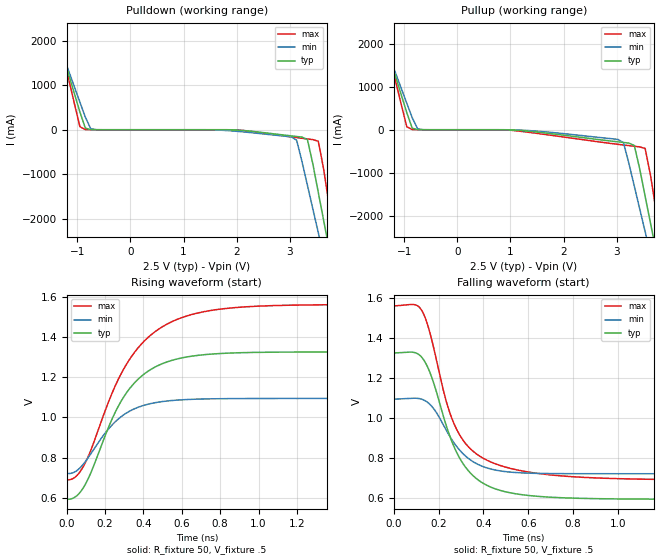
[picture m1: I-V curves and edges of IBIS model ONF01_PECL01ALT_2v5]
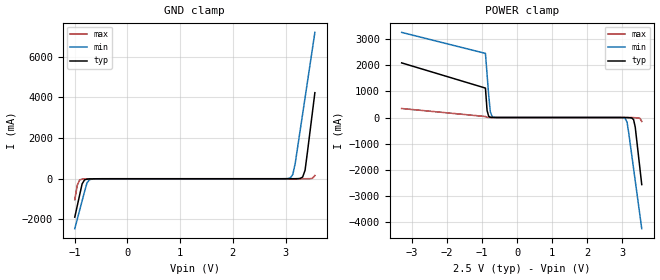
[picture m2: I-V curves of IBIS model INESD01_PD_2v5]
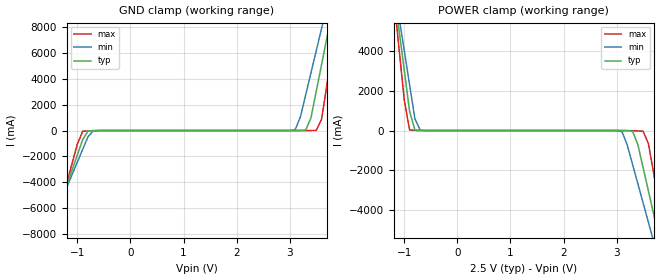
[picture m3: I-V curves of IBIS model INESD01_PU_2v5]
|   This file is an IBIS representation of the   |
|   Integrated Device Technology, Inc.   |
|   8536-02   |
|  Low Skew, 1-to-6, Dual Crystal/LVCMOS-to-3.3V, 2.5V LVPECL Fanout Buffer  |
[IBIS Ver]   4.1
[File name]   8536_02.ibs
[File Rev]   1.0
[Date]   19 Aug 2010
[Source]   Originated at Integrated Device Technology, Inc.
[Disclaimer]
IDT hereby grants the user of this IBIS model a non-exclusive,
nontransferable license to use this IBIS model under the following terms.
Before using this IBIS model, the user should read this license.
If the user does not accept these terms,  the IBIS model should be
returned to IDT within 30 days.
   The user is granted this license only to use the IBIS model and
is not granted rights to sell, load, rent, lease or license the IBIS
model in whole or in part, or in modified form to anyone other than
user. User may modify the IBIS model to suit its specific
applications but rights to derivative works and such modifications
shall belong to IDT.
   This IBIS model is provided on an "AS IS" basis and IDT makes
absolutely no warranty with respect to the information contained
herein. IDT DISCLAIMS AND CUSTOMER WAIVES ALL WARRANTIES, EXPRESS
OR IMPLIED, INCLUDING WARRANTIES OF MERCHANTABILITY OR FITNESS FOR
A PARTICULAR PURPOSE. The entire risk as to quality and performance
is with the Customer. ACCORDINGLY, IN NO EVENT SHALL THE COMPANY BE
LIABLE FOR ANY DAMAGES, WHETHER IN CONTRACT OR TORT,INCLUDING ANY
LOST PROFITS OR OTHER INCIDENTAL, CONSEQUENTIAL, EXEMPLARY, OR
PUNITIVE DAMAGES ARISING OUT OF THE USE OR APPLICATION OF THE IBIS
model provided in this package. Further, IDT reserves the right to
make changes without notice to any product herein to improve
reliability, function, or design. IDT does not convey any license
under patent rights or any other intellectual property rights,
including those of third parties.
   IDT is not obligated to provide maintenance or support
for the licensed IBIS model.
[Copyright]   Copyright 2010 by Integrated Device Technology, Inc.
[Component]   ICS8536G-02
[Manufacturer] Integrated Device Technology, Inc.
[Package]
|TSSOP 24 Lead
|   typ   min   max
R_pkg   60.65m   52.4m   68.9m
L_pkg   1.989nH   1.431nH   2.547nH
C_pkg   0.314pF   0.254pF   0.374pF
[Pin] signal_name  model_name   R_pin   L_pin   C_pin
1   nQ2   ONF01_PECL01ALT   68.9m   2.547n   0.374p
2   Q2   ONF01_PECL01ALT   65.6m   2.323n   0.350p
3   VCC   POWER   62.3m   2.100n   0.326p
4   nQ1   ONF01_PECL01ALT   59.0m   1.877n   0.302p
5   Q1   ONF01_PECL01ALT   55.7m   1.654n   0.278p
6   VEE   GND   52.4m   1.431n   0.254p
7   nQ0   ONF01_PECL01ALT   52.4m   1.431n   0.254p
8   Q0   ONF01_PECL01ALT   55.7m   1.654n   0.278p
9   CLK_SEL0   INESD01_PD   59.0m   1.877n   0.302p
10   XTAL_IN0   NC   62.3m   2.100n   0.326p
11   XTAL_OUT0   NC   65.6m   2.323n   0.350p
12   CLK_EN   INESD01_PU   68.9m   2.547n   0.374p
13   CLK0   INESD02_PD_5V   68.9m   2.547n   0.374p
14   XTAL_IN1   NC   65.6m   2.323n   0.350p
15   XTAL_OUT1   NC   62.3m   2.100n   0.326p
16   CLK_SEL1   INESD01_PD   59.0m   1.877n   0.302p
17   nQ5   ONF01_PECL01ALT   55.7m   1.654n   0.278p
18   Q5   ONF01_PECL01ALT   52.4m   1.431n   0.254p
19   VCC   POWER   52.4m   1.431n   0.254p
20   nQ4   ONF01_PECL01ALT   55.7m   1.654n   0.278p
21   Q4   ONF01_PECL01ALT   59.0m   1.877n   0.302p
22   VCC   POWER   62.3m   2.100n   0.326p
23   nQ3   ONF01_PECL01ALT   65.6m   2.323n   0.350p
24   Q3   ONF01_PECL01ALT   68.9m   2.547n   0.374p
[Diff Pin]  inv_pin  vdiff tdelay_typ tdelay_min  tdelay_max
|Output
2   1   NA   0  0  0
5   4   NA   0  0  0
8   7   NA   0  0  0
18   17   NA   0  0  0
21   20   NA   0  0  0
24   23   NA   0  0  0
[Model Selector] ONF01_PECL01ALT
ONF01_PECL01ALT_2v5  Buffer selection for 2v5
ONF01_PECL01ALT_3v3  Buffer selection for 3v3
[Model Selector] INESD01_PD
INESD01_PD_2v5  Buffer selection for 2v5
INESD01_PD_3v3  Buffer selection for 3v3
[Model Selector] INESD01_PU
INESD01_PU_2v5  Buffer selection for 2v5
INESD01_PU_3v3  Buffer selection for 3v3
[Model Selector] INESD02_PD_5V
INESD02_PD_5V_2v5  Buffer selection for 2v5
INESD02_PD_5V_3v3  Buffer selection for 3v3
| Models and submodels in the file (8): ONF01_PECL01ALT_2v5 (Output_ECL), INESD01_PD_2v5 (Input), INESD01_PU_2v5 (Input), INESD02_PD_5V_2v5 (Input), ONF01_PECL01ALT_3v3 (Output_ECL), INESD01_PD_3v3 (Input), INESD01_PU_3v3 (Input), INESD02_PD_5V_3v3 (Input)
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[Model] ONF01_PECL01ALT_2v5
Model_type  Output_ECL
Polarity   Non-Inverting
Vmeas = .975
Rref = 50
Cref = 0
Vref = .5
|Variable  typ   min   max
C_comp   2p   1.5p   2.5p
[Voltage Range]   2.5   2.375   2.625
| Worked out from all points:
|   rising waveform, R_fixture 50, V_fixture .5: 20-80 % time 228ps typ, 199ps min, 276ps max; typ from 0.592 V to 1.33 V
|   falling waveform, R_fixture 50, V_fixture .5: 20-80 % time 153ps typ, 140ps min, 156ps max; typ from 1.33 V to 0.592 V
| Open source, no load
|  Voltage   I(typ)   I(min)   I(max)
[Pullup]
-3.3V     9.786A     8.425A     12.06A
-1.463V   2.432A     2.308A     2.661A
-952.6mV  398mA      618.5mA    68.87mA
-850.5mV  36.63mA    281.6mA    4.032mA
-646.4mV  229.3uA    964.8uA    177.5uA
3.028V    -282.4mA   -226.8mA   -340.1mA
3.13V     -296.5mA   -301.7mA   -355.4mA
3.334V    -367.3mA   -1.316A    -385.1mA
3.538V    -1.551A    -2.377A    -435.3mA
3.64V     -2.187A    -2.908A    -1.066A
3.844V    -3.46A     -3.969A    -2.688A
6.6V      -20.66A    -18.32A    -24.61A
[Pulldown]
-3.3V     9.786A     8.425A     12.06A
-1.463V   2.432A     2.308A     2.661A
-1.361V   2.024A     1.97A      2.139A
-952.6mV  398mA      618.5mA    68.87mA
-850.5mV  36.63mA    281.6mA    4.032mA
3.028V    -137.6mA   -160.7mA   -160.7mA
3.13V     -151.4mA   -235.1mA   -176.3mA
3.334V    -221.9mA   -1.249A    -206.7mA
3.538V    -1.406A    -2.31A     -257.4mA
3.64V     -2.042A    -2.84A     -888.8mA
3.844V    -3.314A    -3.9A      -2.51A
6.6V      -20.58A    -18.26A    -24.54A
[Ramp]
|   typ   min   max
dV/dt_r   0.586/0.368n   0.299/0.313n   0.698/0.446n
dV/dt_f   0.586/0.258n   0.299/0.226n   0.698/0.290n
R_load =   50.0000
[Rising Waveform]
R_fixture = 50
V_fixture = .5   | VCC_typ - 2V
V_fixture_max = 0.625   | VCC_max - 2V
V_fixture_min = 0.375   | VCC_min - 2V
C_fixture = 0.0p
| Time   typ   min   max
0s        592.5mV    720.8mV    689.3mV
46.2ps    605.5mV    731.1mV    704.8mV
92.4ps    659.4mV    774.5mV    766.4mV
241.5ps   1.003V     967.6mV    1.133V
323.4ps   1.138V     1.029V     1.283V
426.3ps   1.231V     1.066V     1.4V
552.3ps   1.285V     1.084V     1.478V
711.9ps   1.312V     1.092V     1.525V
940.8ps   1.323V     1.094V     1.551V
1.999ns   1.326V     1.094V     1.562V
[Falling Waveform]
R_fixture = 50
V_fixture = .5   | VCC_typ - 2V
V_fixture_max = 0.625   | VCC_max - 2V
V_fixture_min = 0.375   | VCC_min - 2V
C_fixture = 0.0p
0s        1.326V     1.094V     1.562V
92.4ps    1.328V     1.099V     1.568V
123.9ps   1.306V     1.095V     1.541V
168ps     1.209V     1.061V     1.4V
231ps     973.8mV    945.4mV    1.097V
277.2ps   835.9mV    862.7mV    951mV
348.6ps   716.5mV    784.8mV    838.7mV
447.3ps   647.2mV    740.6mV    773mV
865.2ps   596.5mV    720.8mV    701.4mV
1.999ns   592.4mV    720.7mV    689.3mV
[Model] INESD01_PD_2v5
Model_type   Input
Polarity   Non-Inverting
Vinl = 0.8V
Vinh = 2.0V
|   typ   min   max
C_comp   2pF   1.5pF   2.5pF
|   typ   min   max
[Voltage range]  2.5V   2.375V   2.625V
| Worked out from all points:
|   GND clamp passes 1 mA (typ) near -0.55 V on its own axis
|   POWER clamp passes 1 mA (typ) near -0.68 V on its own axis
[GND_clamp]
|Voltage I(typ)   I(min)   I(max)
-1V       -1.886A    -2.451A    -1.028A
-953.5mV  -1.338A    -1.994A    -328mA
-907mV    -789.6mA   -1.537A    -53.04mA
-860.5mV  -251.4mA   -1.081A    -21.51mA
-767.5mV  -17.28mA   -198.8mA   -10.01mA
-674.5mV  -5.28mA    -15.38mA   -3.684mA
3.092V    224.5uA    49.06mA    51.52uA
3.139V    500.8uA    208.3mA    52.98uA
3.185V    1.252mA    774.6mA    56.66uA
3.325V    81.55mA    3.177A     200uA
3.371V    416.9mA    3.978A     464.6uA
3.557V    4.225A     7.185A     159.2mA
[POWER_clamp]
|Voltage   I(typ)   I(min)   I(max)
-3.3V     2.083A     3.246A     343.1mA
-907mV    1.122A     2.445A     37.78mA
-860.5mV  267.5mA    1.644A     5.973mA
-814mV    47.03mA    844mA      1.727mA
-767.5mV  9.66mA     215.3mA    677uA
-674.5mV  960.6uA    12.66mA    131.4uA
3.092V    -1.849mA   -49.09mA   -51.51uA
3.139V    -3.491mA   -186mA     -159.7uA
3.325V    -84.03mA   -1.955A    -5.102mA
3.371V    -365.4mA   -2.411A    -8.31mA
3.51V     -2.01A     -3.782A    -35.44mA
3.557V    -2.558A    -4.239A    -152.3mA
[Model] INESD01_PU_2v5
Model_type   Input
Polarity   Non-Inverting
Vinl = 1.4V
Vinh = 1.85V
|   typ   min   max
C_comp   2pF   1.5pF   2.5pF
|   typ   min   max
[Voltage range]  2.5V   2.375V   2.625V
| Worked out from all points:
|   GND clamp passes 1 mA (typ) near -0.54 V on its own axis
|   POWER clamp passes 1 mA (typ) near -0.66 V on its own axis
[GND_clamp]
|Voltage   I(typ)   I(min)   I(max)
-2.5V     -19.6A     -17.18A    -23.67A
-1.6V     -8.969A    -8.332A    -10.1A
-1.5V     -7.788A    -7.349A    -8.588A
-900mV    -707.1mA   -1.46A     -57.43mA
-700mV    -7.027mA   -24.05mA   -13.28mA
3.1V      199.2uA    53.94mA    11.78uA
3.3V      28.4mA     2.748A     652.4uA
3.5V      3.045A     6.192A     15.72mA
3.6V      5.115A     7.914A     872.4mA
3.7V      7.185A     9.638A     3.52A
3.9V      11.33A     13.09A     8.818A
5V        34.14A     32.07A     37.99A
[POWER_clamp]
|Voltage   I(typ)   I(min)   I(max)
-1.5V     9.257A     9.207A     9.48A
-1.2V     7.185A     7.484A     6.83A
-1.1V     5.115A     5.761A     4.182A
-900mV    976.9mA    2.318A     34.23mA
-700mV    1.582mA    24.31mA    1.044mA
3.1V      -2.107mA   -51.03mA   -534.5uA
3.3V      -35.62mA   -1.705A    -10.86mA
3.5V      -1.886A    -3.666A    -39.41mA
3.6V      -3.066A    -4.647A    -666.9mA
3.8V      -5.426A    -6.612A    -3.684A
3.9V      -6.607A    -7.595A    -5.193A
5V        -19.6A     -18.41A    -21.79A
